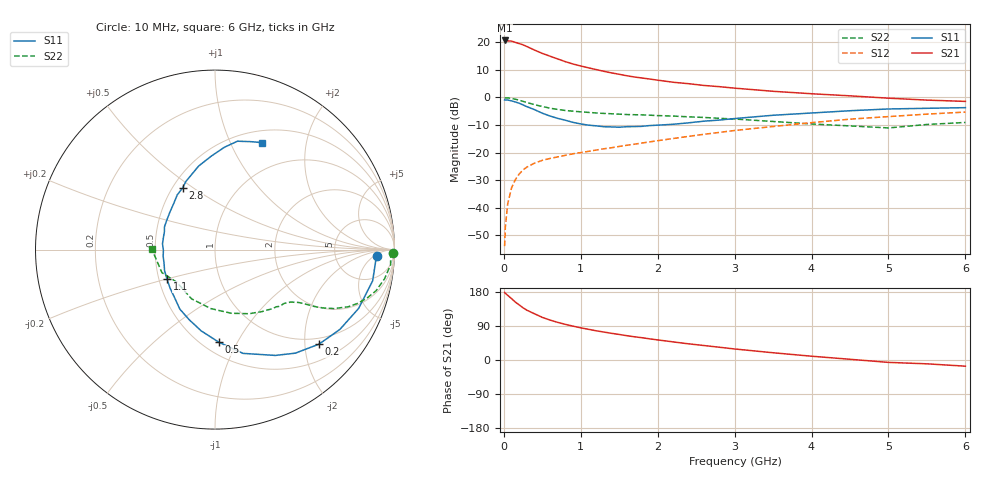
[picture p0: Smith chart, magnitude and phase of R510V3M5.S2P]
! SIEMENS Small Signal Semiconductors
! BFR183
! Si NPN RF Bipolar Junction Transistor in SOT23
! VCE = 10 V  IC = 3.5 mA
! Common Emitter S-Parameters:  May  1996
# GHz  S  MA  R  50
!  f  S11  S21  S12  S22
! GHz  MAG  ANG  MAG  ANG  MAG  ANG  MAG  ANG
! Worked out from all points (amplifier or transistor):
!   36 points, 10 MHz to 6 GHz, reference 50 ohm
!   highest |S21| = 20.7 dB at 10 MHz (marker M1)
!   |S21| within 3 dB of that: start of sweep to 361.3 MHz
!   unconditionally stable (mu >= 1): 1.247 GHz to 2.825 GHz
!   at 250 MHz: K = 0.32, MSG = 22.7 dB, |S12| = -26.3 dB
!   at 1.4 GHz: K = 1.04, MAG = 12.3 dB, |S12| = -18.3 dB
!   at 6 GHz: K = 0.87, MSG = 1.9 dB, |S12| = -5.3 dB
!   S11 on the Smith chart (normalised r, x): 10 MHz: 17, -6; 200 MHz: 0.85, -2.32; 500 MHz: 0.60, -0.84; 1.1 GHz: 0.55, -0.20; 2.8 GHz: 0.56, +0.45; 6 GHz: 0.64, +1.33
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0.01  0.9019 -2.2  10.79 178.1  0.002 87.1  0.9905 -1.0
0.02  0.8971 -4.4  10.78 175.9  0.0045 84.1  0.9798 -2.0
0.05  0.8955 -11.2  10.62 170.7  0.0117 83.7  0.9819 -5.0
0.1  0.8646 -22.3  10.49 162.0  0.0228 77.9  0.9584 -9.8
0.15  0.8258 -32.6  9.949 152.8  0.0323 72.5  0.9263 -14.3
0.2  0.783 -42.3  9.466 145.3  0.0408 67.4  0.8901 -17.6
0.25  0.7302 -52.2  8.992 137.7  0.0483 63.6  0.8469 -20.8
0.3  0.6788 -60.3  8.37 131.4  0.0545 61.0  0.806 -23.3
0.4  0.5989 -74.9  7.21 121.8  0.0642 56.3  0.739 -26.4
0.5  0.5165 -87.6  6.284 112.5  0.0721 53.7  0.6831 -28.4
0.6  0.4595 -99.6  5.594 105.4  0.078 52.3  0.6377 -29.8
0.7  0.4163 -110.2  4.983 99.3  0.0833 51.7  0.6049 -30.6
0.8  0.3851 -120.6  4.448 94.0  0.0889 51.5  0.5786 -31.4
0.9  0.352 -129.3  4.03 89.3  0.095 51.4  0.5621 -31.9
1.1  0.3137 -148.6  3.442 81.0  0.105 52.3  0.5342 -33.4
1.6  0.2945 173.6  2.467 64.1  0.1355 54.8  0.4888 -37.8
2.2  0.3255 141.0  1.884 47.8  0.1793 55.3  0.4584 -46.0
2.8  0.3878 117.7  1.566 33.7  0.2315 52.9  0.4175 -57.2
3.5  0.4742 101.1  1.29 19.1  0.2965 47.1  0.3658 -75.8
4.5  0.573 84.7  1.067 1.9  0.403 36.4  0.3037 -115.6
5.5  0.6341 71.5  0.893 -10.1  0.4973 23.9  0.3225 -156.6
6  0.6515 66.1  0.846 -16.3  0.5419 15.7  0.3514 179.7
